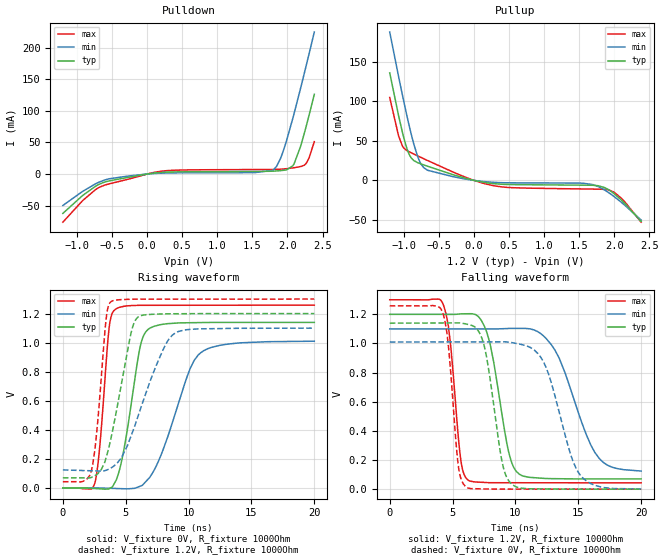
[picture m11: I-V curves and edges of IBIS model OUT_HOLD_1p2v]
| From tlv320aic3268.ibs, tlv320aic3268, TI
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|   OUT_HOLD_1p2v
[Model]   OUT_HOLD_1p2v
Model_type   Output
Polarity   Non-Inverting
Vmeas = 0.6
Vref = 0
Cref = 5pF
Rref = 10000
|   typ   min   max
C_comp   1.444pF   1.430pF   1.479pF
[Voltage Range]   1.2   1.1   1.3
[Temperature Range]   27   125   -40
[Pullup Reference]   1.2   1.1   1.3
[Pulldown Reference]   -0   -0   -0
[Power Clamp Reference]   1.2   1.1   1.3
[GND Clamp Reference]   -0   -0   -0
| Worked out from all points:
|   slope of the pulldown table from 0 to 0.18 V, typ, clamps not added: 75.4 ohm
|   slope of the pullup table from 0 to 0.18 V, typ, clamps not added: 60.3 ohm
|   falling waveform, V_fixture 1.2V, R_fixture 1000Ohm: 20-80 % time 1.32ns typ, 2.46ns min, 764ps max; typ from 1.2 V to 0.07 V
|   rising waveform, V_fixture 0V, R_fixture 1000Ohm: 20-80 % time 1.24ns typ, 2.37ns min, 675ps max; typ from 0 V to 1.14 V
|   rising waveform, V_fixture 1.2V, R_fixture 1000Ohm: 20-80 % time 1.5ns typ, 2.48ns min, 731ps max; typ from 0.07 V to 1.2 V
|   falling waveform, V_fixture 0V, R_fixture 1000Ohm: 20-80 % time 1.16ns typ, 1.98ns min, 704ps max; typ from 1.14 V to 0 V
[Pulldown]
|   Voltage   I(typ)   I(min)   I(max)
-1.2V     -62.24mA   -49.71mA   -76.11mA
-912mV    -33.39mA   -26.97mA   -41.4mA
-696mV    -16.88mA   -13.38mA   -21.88mA
42mV      709.1uA    401.2uA    1.225mA
420mV     3.452mA    1.927mA    6.193mA
1.788V    4.529mA    5.894mA    7.322mA
1.842V    4.902mA    11.83mA    7.438mA
1.914V    5.586mA    28.51mA    7.82mA
2.094V    16.24mA    95.7mA     10.05mA
2.184V    42.94mA    134.6mA    11.79mA
2.274V    78.76mA    174.9mA    18.19mA
2.382V    126.1mA    224.6mA    51.31mA
[Pullup]
|   Voltage   I(typ)   I(min)   I(max)
-1.2V     136.2mA    187.8mA    105mA
-1.074V   82.05mA    131.6mA    56.37mA
-1.02V    61.18mA    108.4mA    43.65mA
-948mV    38.49mA    78.97mA    37.34mA
-894mV    28.42mA    58.56mA    34.89mA
-804mV    22.51mA    30.65mA    31.11mA
-714mV    19.52mA    15.97mA    27.36mA
-300mV    7.232mA    4.735mA    10.61mA
294mV     -4.236mA   -2.564mA   -6.927mA
1.77V     -6.792mA   -7.864mA   -11.12mA
2.004V    -17.41mA   -21.04mA   -15.6mA
2.382V    -52.11mA   -50.35mA   -52.99mA
[Ramp]
R_load = 1000
|   typ   min   max
dV/dt_r   0.683698/1.24067e-009  0.605149/2.37057e-009  0.754921/6.75347e-010
dV/dt_f   0.67794/1.32258e-009  0.585387/2.46377e-009   0.75409/7.64287e-010
[Falling Waveform]
V_fixture = 1.2V
V_fixture_min = 1.1V
V_fixture_max = 1.3V
R_fixture = 1000Ohm
C_fixture = 0F
|   Time   V(typ)   V(min)   V(max)
0s        1.2V       1.1V       1.3V
4.237ns   1.2V       1.1V       1.271V
4.864ns   1.2V       1.1V       973.1mV
5.655ns   1.203V     1.1V       199.9mV
6.22ns    1.204V     1.1V       62.8mV
7.713ns   1.079V     1.1V       45.32mV
10.08ns   120.7mV    1.103V     44.12mV
13.13ns   72.02mV    956.3mV    43.83mV
16.65ns   70.25mV    212.2mV    43.5mV
20ns      70.1mV     124.3mV    43.18mV
[Rising Waveform]
V_fixture = 0V
V_fixture_min = 0V
V_fixture_max = 0V
R_fixture = 1000Ohm
C_fixture = 0F
|   Time   V(typ)   V(min)   V(max)
0s        -748.4nV   1.348mV    4.699nV
2.541ns   -3.5mV     738.3uV    32.27mV
2.942ns   -5.723mV   138.3uV    291.4mV
3.691ns   -4.626mV   -1.877mV   1.108V
4.185ns   45.26mV    -3.207mV   1.23V
4.83ns    252.4mV    -4.946mV   1.25V
6.11ns    955.8mV    11.01mV    1.257V
6.824ns   1.094V     64.85mV    1.257V
10.98ns   1.138V     931.5mV    1.257V
20ns      1.139V     1.01V      1.258V
[Rising Waveform]
V_fixture = 1.2V
V_fixture_min = 1.1V
V_fixture_max = 1.3V
R_fixture = 1000Ohm
C_fixture = 0F
|   Time   V(typ)   V(min)   V(max)
0s        70.1mV     124.6mV    43.18mV
2.251ns   72.64mV    118.5mV    112.4mV
2.7ns     93.44mV    117.3mV    389.2mV
3.417ns   202mV      121.6mV    1.144V
3.82ns    340.1mV    137.3mV    1.281V
5.427ns   1.067V     358.8mV    1.299V
6.022ns   1.178V     504.8mV    1.299V
7.959ns   1.198V     948.5mV    1.299V
9.084ns   1.199V     1.073V     1.299V
20ns      1.2V       1.1V       1.3V
[Falling Waveform]
|Gnd
V_fixture = 0V
V_fixture_min = 0V
V_fixture_max = 0V
R_fixture = 1000Ohm
C_fixture = 0F
|   Time   V(typ)   V(min)   V(max)
0s        1.139V     1.01V      1.258V
4.185ns   1.141V     1.01V      1.217V
4.671ns   1.141V     1.011V     982.3mV
5.453ns   1.141V     1.011V     163mV
6.06ns    1.134V     1.011V     15.79mV
7.525ns   980.3mV    1.011V     1.507mV
9.64ns    40.06mV    1.007V     546.5uV
12.22ns   1.755mV    874.7mV    410.1uV
15.23ns   179uV      88.62mV    251.6uV
20ns      -433.3nV   1.316mV    3.556nV
